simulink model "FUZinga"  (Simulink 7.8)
settings: Solver=ode45  StartTime=0.0  StopTime=30  FixedStep=0.1  RelTol=1e-3
undefined symbols (not defined in the file or in its folder): deg, kg, m, N, s
libraries: mblibv1 x5, fuzblock x1

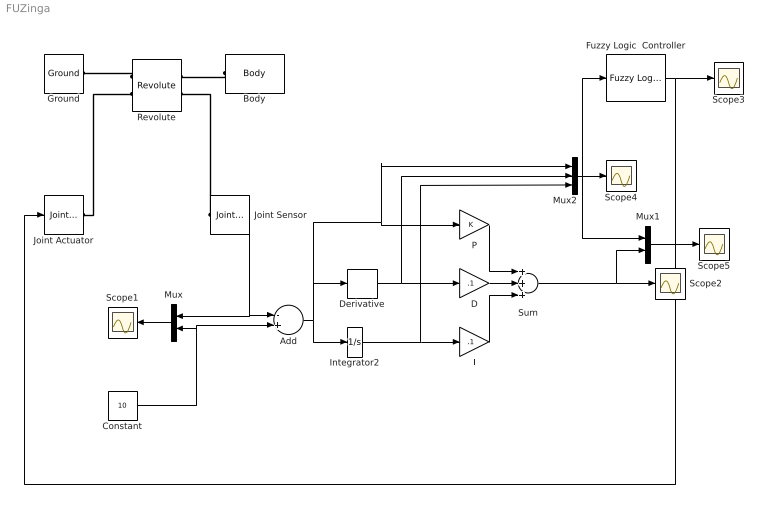
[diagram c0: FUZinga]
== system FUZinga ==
  Add : Sum  Inputs=-+
  Body : mblibv1/Bodies/Body  LConnTagsString=CS1  UpdateFromCAD=off  DialogClass=MechanicalBodyBlock  Mass=1  MassUnits=kg  InertiaUnits=kg*m^2  Inertia=eye(3)  Shape=Cylinder  ShapeDims=[1 1]  ShapeUnits=m  ShapeUse=false  Density=1  DensityUnits=kg/m^3  DensityUse=false  GraphicsMode=MACHINE_DEFAULT  BodyColorSelMode=MACHINE_DEFAULT  BodyColor=[1 0 0]  AttachedToCS=CG  CG=Left$CG$[0 -0.5 0]$WORLD$WORLD$m$[0 0 0]$Euler X-Y-Z$deg$WORLD$false$none  WorkingFrames=Left$CS1$[0 0.5 0]$CG$CG$m$[0 0 0]$Euler X-Y-Z$deg$WORLD$true$none#Right$CS2$[0 -0.5 0]$CG$CG$m$[0 0 0]$Euler X-Y-Z$deg$WORLD$false$none  CGPos=[0 -0.5 0]  CGRot=[0 0 0]  CS0Pos=[]  CS0Rot=[]  CS1Pos=[0 0.5 0]  CS1Rot=[0 0 0]  CS2Pos=[0 -0.5 0]  CS2Rot=[0 0 0]  CS3Pos=[]  CS3Rot=[]  CS4Pos=[]  CS4Rot=[]  CS5Pos=[]  CS5Rot=[]  CS6Pos=[]  CS6Rot=[]  CS7Pos=[]  CS7Rot=[]  CS8Pos=[]  CS8Rot=[]  CS9Pos=[]  CS9Rot=[]  CS10Pos=[]  CS10Rot=[]  CS11Pos=[]  CS11Rot=[]  CS12Pos=[]  CS12Rot=[]  CS13Pos=[]  CS13Rot=[]  CS14Pos=[]  CS14Rot=[]  CS15Pos=[]  CS15Rot=[]  CS16Pos=[]  CS16Rot=[]  CS17Pos=[]  CS17Rot=[]  CS18Pos=[]  CS18Rot=[]  CS19Pos=[]  CS19Rot=[]  CS20Pos=[]  CS20Rot=[]
  Constant : Constant  Value=10
  D : Gain  Gain=.1
  Derivative : Derivative
  Fuzzy Logic  Controller : fuzblock/Fuzzy Logic  Controller  fis=inga
  Ground : mblibv1/Bodies/Ground  UpdateFromCAD=off  LeftPortType=env  RightPortType=workingframe  PhysicalDomain=Mechanical  DialogClass=GroundBlock  CoordPosition=[0 0 0]  CoordPositionUnits=m  StateVectorMgrId=0  MachineId=[1 0]  ShowEnvPort=off
  I : Gain  Gain=.1
  Integrator2 : Integrator
  Joint Actuator : mblibv1/Sensors &  Actuators/Joint Actuator  UpdateFromCAD=off  PhysicalDomain=Mechanical  PortType=blob  ActuationStyle=Force  AngleUnits=deg  ArcVelocityUnits=deg/s  ArcAccelerationUnits=deg/s^2  CoordPositionUnits=m  VelocityUnits=m/s  AccelerationUnits=m/s^2  ForceUnits=N  TorqueUnits=N*m  ActiveIO=on  Width=1  DialogClass=MechanicalActuatorBlock  Primitive=R1  ReferenceFrame=Absolute (World)
  Joint Sensor : mblibv1/Sensors &  Actuators/Joint Sensor  UpdateFromCAD=off  PhysicalDomain=Mechanical  PortType=blob  Muxed=on  Pose=off  Angle=on  AngleUnits=deg  ArcVelocity=off  ArcVelocityUnits=deg/s  ArcAcceleration=off  ArcAccelerationUnits=deg/s^2  CoordPosition=on  CoordPositionUnits=m  Velocity=off  VelocityUnits=m/s  Acceleration=off  AccelerationUnits=m/s^2  Quaternion=on  QuaternionDT=off  QuaternionDDT=off  QuaternionUnits=off  OutputVector=[1]  ActiveIO=on  Width=1  DialogClass=MechanicalSensorBlock  Primitive=R1  Force=off  ForceUnits=N  Torque=off  TorqueUnits=N*m  ReferenceFrame=Absolute (World)  ReactionSensedSide=Base  ReactionReferenceFrame=Absolute (World)  ReactionForce=off  ReactionForceUnits=N  ReactionMoment=off  ReactionMomentUnits=N*m
  Mux : Mux  Inputs=2
  Mux1 : Mux  Inputs=2
  Mux2 : Mux  Inputs=3
  P : Gain
  Revolute : mblibv1/Joints/Revolute  LConnTagsString=__newl0|SA1  RConnTagsString=__newr0|SA1  UpdateFromCAD=off  NumSAPorts=2  CutJoint=off  MarkAsCut=off  Primitives=prismatic  PrimitiveProps=R1$World$[0 0 1]$revolute  DialogClass=JointBlock  R1Axis=[0 0 1]
  Scope{1..5} (5 alike) : Scope
  Sum : Sum  Inputs=+++
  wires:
  Joint Sensor/1 -> Add/1, Mux/1
  Mux/1 -> Scope1/1
  Integrator2/1 -> I/1, Mux2/3
  Add/1 -> Derivative/1, P/1, Mux2/1, Integrator2/1
  Derivative/1 -> D/1, Mux2/2
  Constant/1 -> Add/2, Mux/2
  Mux2/1 -> Scope4/1, Mux1/1, Fuzzy Logic  Controller/1
  P/1 -> Sum/1
  D/1 -> Sum/2
  I/1 -> Sum/3
  Sum/1 -> Scope2/1, Mux1/2
  Mux1/1 -> Scope5/1
  Fuzzy Logic  Controller/1 -> Scope3/1, Joint Actuator/1
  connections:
  Revolute/LConn1 -- Ground/RConn1
  Body/LConn1 -- Revolute/RConn1
  Joint Actuator/RConn1 -- Revolute/LConn2
  Joint Sensor/LConn1 -- Revolute/RConn2
